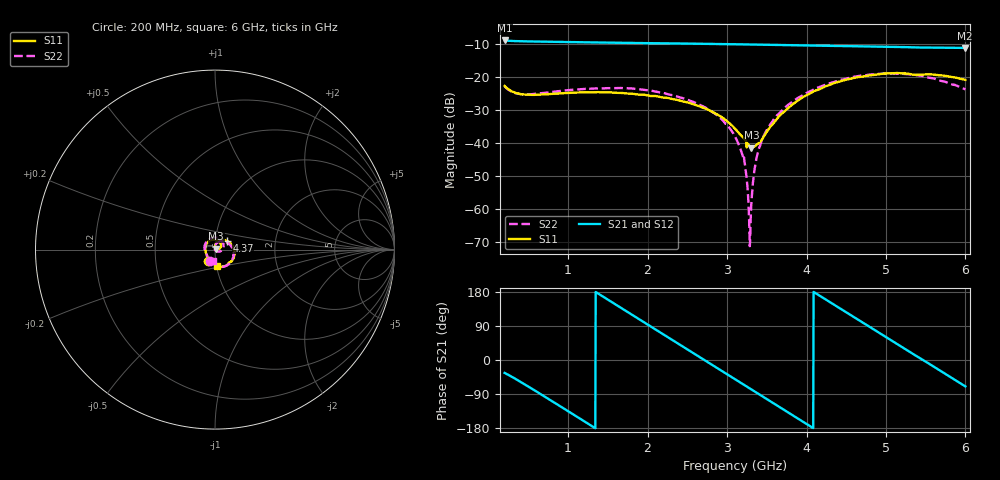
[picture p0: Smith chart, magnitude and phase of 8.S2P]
!Agilent Technologies,E5071C,MY46316741,A.11.02
!Date: Fri Apr 15 16:20:10 2022
!Data & Calibration Information:
!Freq	S11:SOLT2(ON)	S21:SOLT2(ON)	S12:SOLT2(ON)	S22:SOLT2(ON)
!PortZ  Port1:50+j0  Port2:50+j0
!Above PortZ is port z conversion or system Z0 setting when saving the data.
!When reading, reference impedance value at option line is always used.
# Hz S dB R 50
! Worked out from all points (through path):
!   1200 points, 200 MHz to 6 GHz, reference 50 ohm
!   highest |S21| = -9.01 dB at 200 MHz (marker M1); lowest = -11.3 dB at 5.99 GHz (marker M2)
!   group delay of S21, straight-line fit = 364 ps
!   lowest |S11| = -41.4 dB at 3.306 GHz (marker M3), VSWR 1.02, Z = 50.7 + j0.517 ohm
!   |S11| at or under -10 dB: start of sweep to end of sweep
!   |S22| runs from -71.2 to -19.0 dB; largest |S21 - S12| = 0.001
!   S11 on the Smith chart (normalised r, x): 200 MHz: 0.92, -0.12; 4.37 GHz: 1.13, +0.11; 6 GHz: 1.01, -0.18
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2e8  -22.76 -120.3  -9.01 -34.1  -9.02 -34.1  -22.88 -113.3
6.885738e8  -25.32 178.8  -9.39 -94.5  -9.39 -94.5  -24.91 -176.0
1.167473e9  -24.72 137.5  -9.56 -157.1  -9.56 -157.1  -23.73 135.7
1.578649e9  -24.81 104.6  -9.71 149.0  -9.71 149.0  -23.43 96.1
2.134946e9  -25.97 62.9  -9.86 76.1  -9.86 76.2  -24.64 40.5
2.739616e9  -29.72 20.2  -10.04 -3.3  -10.04 -3.3  -29.47 -14.3
3.102419e9  -35.72 8.1  -10.17 -51.0  -10.17 -50.9  -38.14 -46.9
3.204003e9  -38.40 13.2  -10.20 -64.4  -10.21 -64.3  -44.42 -58.3
3.237865e9  -39.39 19.9  -10.22 -68.8  -10.22 -68.7  -48.94 -59.5
3.271726e9  -40.64 28.0  -10.23 -73.3  -10.23 -73.2  -59.30 -70.9
3.305588e9  -41.37 36.6  -10.24 -77.7  -10.25 -77.6  -58.10 128.9
3.334612e9  -41.21 45.6  -10.25 -81.5  -10.26 -81.4  -50.04 116.5
3.368474e9  -40.63 58.5  -10.27 -86.0  -10.27 -85.9  -44.88 110.2
3.479733e9  -37.41 82.3  -10.31 -100.5  -10.31 -100.5  -36.99 101.1
3.731276e9  -30.24 84.7  -10.41 -133.5  -10.41 -133.5  -29.22 77.7
4.069892e9  -24.65 61.6  -10.56 -177.8  -10.56 -177.7  -24.10 47.3
4.369808e9  -21.71 37.8  -10.67 143.0  -10.67 143.1  -21.37 20.6
4.703586e9  -19.89 9.6  -10.80 99.3  -10.80 99.4  -19.56 -8.7
5.037364e9  -18.95 -17.2  -10.93 55.7  -10.93 55.9  -19.05 -37.5
5.511426e9  -19.26 -50.4  -11.16 -5.7  -11.16 -5.6  -20.07 -74.0
5.990325e9  -20.87 -82.1  -11.27 -68.4  -11.28 -68.4  -23.69 -97.3
6e9  -20.93 -82.5  -11.27 -69.7  -11.28 -69.6  -23.78 -97.4
